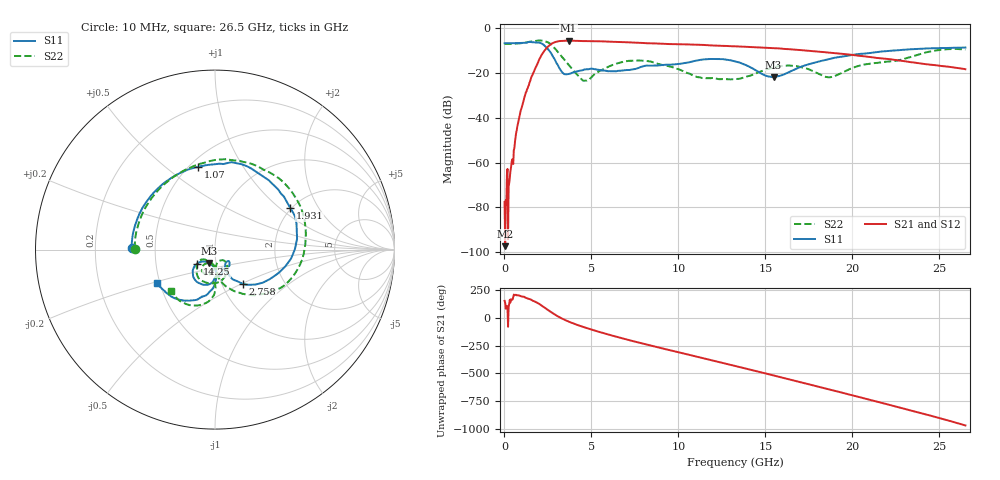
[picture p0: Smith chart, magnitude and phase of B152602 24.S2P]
!  2-Port S-parameters saved by WinCal
! VAR MeasName=S-Parameters (CALIBRATED_DATA) read from VNA (N5242A)
! VAR MeasDate=2016-1-5 16:28:41
! VAR NAME=B152602 24
! VAR FILENAME=B152602 24.S2P
! VAR DATE=2016-1-5 16:28:41
! VAR PHYS_PORTS=1,2
# Hz S DB R 50
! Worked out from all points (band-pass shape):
!   801 points, 10 MHz to 26.5 GHz, reference 50 ohm
!   highest |S21| = -5.51 dB at 3.685 GHz (marker M1); lowest = -97.4 dB at 43.11 MHz (marker M2)
!   |S21| within 3 dB of the highest: 2.457 GHz to 14.62 GHz (12.17 GHz wide, 142 % of centre)
!   lowest |S11| = -21.8 dB at 15.47 GHz (marker M3), VSWR 1.18, Z = 46.3 - j6.95 ohm
!   |S11| at or under -10 dB: 2.58 GHz to 22.23 GHz (19.65 GHz wide, 158 % of centre)
!   |S22| runs from -23.4 to -5.4 dB; largest |S21 - S12| = 0.003
!   S11 on the Smith chart (normalised r, x): 10 MHz: 0.36, +0.01; 1.07 GHz: 0.55, +0.65; 1.931 GHz: 1.98, +1.19; 2.758 GHz: 1.25, -0.51; 14.25 GHz: 0.81, -0.13; 26.5 GHz: 0.48, -0.21
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1e7  -6.65 179.2  -77.69 152.7  -68.31 41.2  -6.97 179.3
4.31125e7  -6.65 176.9  -97.41 133.2  -76.66 106.8  -6.98 177.4
1.755625e8  -6.64 167.1  -62.86 86.8  -63.05 91.9  -6.95 169.2
3.41125e8  -6.64 155.0  -64.01 136.5  -64.58 139.3  -6.93 159.0
7.38475e8  -6.61 125.9  -43.99 -157.9  -44.09 -157.5  -6.79 134.3
1.0696e9  -6.54 101.5  -33.44 -169.9  -33.45 -169.9  -6.53 113.2
1.930525e9  -6.39 28.8  -15.30 130.7  -15.30 130.8  -5.46 47.8
2.758338e9  -12.16 -50.7  -6.65 42.8  -6.64 42.8  -7.80 -33.5
3.685488e9  -20.43 -42.9  -5.51 -33.9  -5.51 -33.9  -16.25 -83.6
4.447075e9  -18.80 -46.0  -5.68 -78.4  -5.67 -78.4  -22.89 -79.2
6.50005e9  -19.02 -69.5  -6.08 -173.1  -6.08 -173.1  -15.64 -72.3
8.851038e9  -16.59 -84.8  -6.80 93.5  -6.77 93.4  -15.94 -129.6
1.106958e10  -14.37 -97.5  -7.30 9.6  -7.28 9.7  -21.75 -138.7
1.3255e10  -14.78 -132.6  -8.04 -72.7  -8.02 -72.9  -22.70 -110.0
1.424838e10  -17.88 -141.9  -8.40 -110.9  -8.36 -110.9  -20.83 -96.0
1.547354e10  -21.78 -113.9  -8.88 -158.2  -8.85 -158.2  -17.43 -99.8
1.769208e10  -15.61 -88.0  -10.15 114.5  -10.11 114.7  -18.99 -126.6
1.868545e10  -13.73 -91.6  -10.86 75.4  -10.86 75.1  -21.88 -106.7
1.994372e10  -11.94 -99.7  -11.83 25.3  -11.82 25.2  -17.88 -84.5
2.209604e10  -10.10 -114.8  -13.76 -61.0  -13.69 -61.2  -14.89 -92.0
2.43808e10  -8.95 -132.3  -16.17 -154.6  -16.13 -155.1  -10.51 -98.7
2.65e10  -8.58 -150.3  -18.27 112.4  -18.27 111.9  -9.49 -136.7
